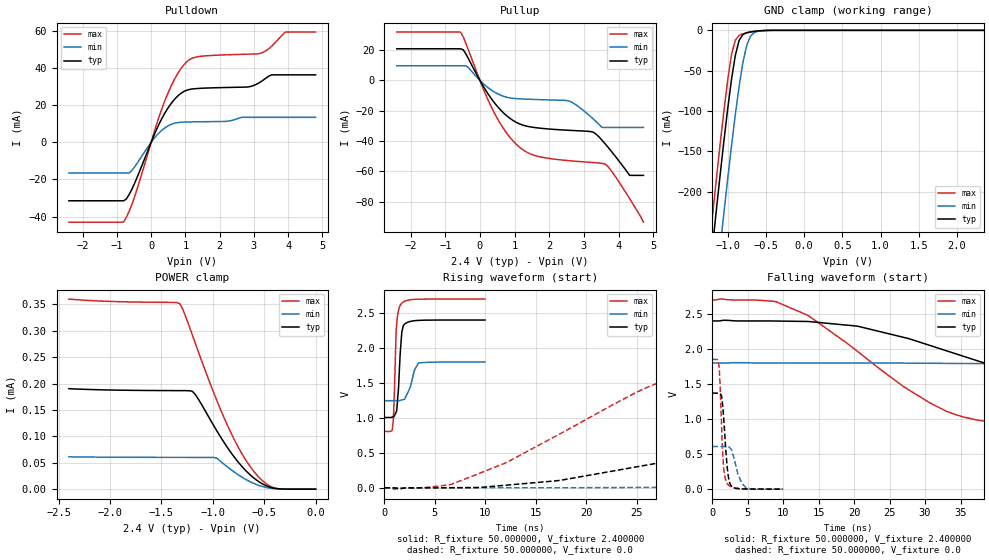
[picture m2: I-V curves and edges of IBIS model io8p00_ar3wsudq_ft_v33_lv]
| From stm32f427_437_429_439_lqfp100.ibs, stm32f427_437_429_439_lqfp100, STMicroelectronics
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|   Model io8p00_ar3wsudq_ft_v33_lv
[Model]  io8p00_ar3wsudq_ft_v33_lv
Model_type I/O
Polarity   Non-Inverting
Enable   Active-Low
Vinl =   0.720000V
Vinh =   1.680000V
Vmeas =  1.200000V
Cref =   50.000000pF
Rref =   100.000000M
Vref =   0.0V
C_comp   3.737300pF   3.690400pF   3.817400pF
[Temperature Range]   25.000000   0.125000k   -40.000000
[Pullup Reference]   2.400000V   1.800000V   2.700000V
[Pulldown Reference]   0.0V   0.0V   0.0V
[POWER Clamp Reference]   2.400000V   1.800000V   2.700000V
[GND Clamp Reference]   0.0V   0.0V   0.0V
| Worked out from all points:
|   slope of the pulldown table from 0 to 0.36 V, typ, clamps not added: 25 ohm
|   slope of the pullup table from 0 to 0.36 V, typ, clamps not added: 27.7 ohm
|   GND clamp passes 1 mA (typ) near -0.62 V on its own axis
|   rising waveform, R_fixture 50.000000, V_fixture 2.400000: 20-80 % time 349ps typ, 698ps min, 263ps max; typ from 1.01 V to 2.4 V
|   rising waveform, R_fixture 50.000000, V_fixture 0.0: 20-80 % time 30.9ns typ, 81.7ns min, 14.6ns max; typ from 0 V to 1.37 V
|   falling waveform, R_fixture 50.000000, V_fixture 2.400000: 20-80 % time 28.7ns typ, 81ns min, 15.9ns max; typ from 2.4 V to 1.01 V
|   falling waveform, R_fixture 50.000000, V_fixture 0.0: 20-80 % time 600ps typ, 1.08ns min, 461ps max; typ from 1.37 V to 0 V
[Pulldown]
|Voltage   I(typ)   I(min)   I(max)
-2.4V     -31.47mA   -16.45mA   -43.01mA
-800mV    -31.47mA   -16.45mA   -42.85mA
-480mV    -21.98mA   -13.17mA   -29.21mA
80mV      3.63mA     1.966mA    5.014mA
480mV     18.16mA    8.738mA    26.02mA
800mV     25.38mA    10.72mA    37.77mA
1.12V     28.53mA    11.02mA    44.6mA
2.8V      29.84mA    13.49mA    47.53mA
3.2V      32.65mA    13.49mA    48.04mA
3.52V     36.4mA     13.49mA    51.83mA
3.92V     36.4mA     13.49mA    59.44mA
4.8V      36.4mA     13.49mA    59.44mA
[Pullup]
|Voltage   I(typ)   I(min)   I(max)
-2.4V     20.89mA    9.661mA    31.89mA
-560mV    20.89mA    9.661mA    31.89mA
-400mV    17.28mA    9.661mA    24.06mA
320mV     -11.75mA   -6.207mA   -17.08mA
640mV     -20.52mA   -10.1mA    -30.35mA
960mV     -26.47mA   -11.82mA   -40.02mA
1.52V     -30.88mA   -12.51mA   -49.05mA
2.56V     -32.88mA   -13.52mA   -52.9mA
3.28V     -34.25mA   -25.62mA   -54.18mA
3.6V      -41.44mA   -30.99mA   -55.03mA
4.32V     -62.62mA   -30.99mA   -77.98mA
4.72V     -62.62mA   -30.99mA   -93.5mA
[GND_clamp]
|Voltage   I(typ)   I(min)   I(max)
-2.4V     -1.437A    -1.518A    -1.411A
-1.25V    -315.9mA   -407.2mA   -278.2mA
-1.2V     -270.1mA   -361.3mA   -232.1mA
-1.15V    -225mA     -316mA     -186.8mA
-1.1V     -180.9mA   -271.3mA   -142.7mA
-1.05V    -138.2mA   -227.5mA   -100.5mA
-950mV    -61.14mA   -143.6mA   -30.43mA
-900mV    -31.23mA   -104.7mA   -12.14mA
-850mV    -12.49mA   -69.4mA    -6.221mA
-750mV    -2.898mA   -18.35mA   -3.18mA
-600mV    -750.2uA   -1.218mA   -738.3uA
2.35V     0A         0A         0A
[POWER_clamp]
|Voltage   I(typ)   I(min)   I(max)
-2.4V     190.2uA    61.19uA    359.9uA
-1.32V    186.6uA    60.14uA    351.2uA
-1.29V    186.5uA    60.13uA    339.6uA
-1.2V     185.4uA    60.11uA    292.6uA
-1.17V    179.2uA    60.11uA    276.3uA
-960mV    110.2uA    58.62uA    167.5uA
-870mV    82.44uA    43.99uA    126.3uA
-750mV    50.58uA    26.92uA    78.64uA
-630mV    25.94uA    13.41uA    41.02uA
-510mV    9.22uA     4.527uA    14.97uA
-420mV    2.425uA    1.38uA     3.75uA
0V        0A         0A         0A
[Ramp]
| variable   typ   min   max
dV/dt_r  0.82266/30.92657n   0.36308/83.78730n   1.11084/14.58848n
dV/dt_f  0.83688/28.73017n   0.32688/81.44683n   1.13728/15.90715n
R_load = 50.000000
[Rising Waveform]
R_fixture= 50.000000
V_fixture= 2.400000
V_fixture_min= 1.800000
V_fixture_max= 2.700000
|time   V(typ)   V(min)   V(max)
0s        1.006V     1.247V     804.6mV
780.8ps   1.011V     1.247V     840.7mV
880.9ps   1.015V     1.247V     966.7mV
1.181ns   1.09V      1.247V     2.284V
1.381ns   1.4V       1.246V     2.53V
1.642ns   2.075V     1.253V     2.628V
1.722ns   2.226V     1.256V     2.64V
1.882ns   2.323V     1.262V     2.659V
3.383ns   2.395V     1.786V     2.699V
9.97ns    2.4V       1.8V       2.7V
[Rising Waveform]
R_fixture= 50.000000
V_fixture= 0.0
V_fixture_min= 0.0
V_fixture_max= 0.0
|time   V(typ)   V(min)   V(max)
0s        9.861nV    351.5nV    28.52nV
7.007ns   1.54mV     -65.12uV   70.14mV
12.01ns   36.61mV    -30.31uV   355mV
17.02ns   99.51mV    83.56uV    742.1mV
28.03ns   377mV      6.556mV    1.543V
39.04ns   686.7mV    29.19mV    1.767V
56.56ns   1.125V     88.61mV    1.83V
77.58ns   1.308V     182.7mV    1.85V
153.2ns   1.369V     510.1mV    1.852V
249.2ns   1.37V      609.1mV    1.852V
[Falling Waveform]
R_fixture= 50.000000
V_fixture= 2.400000
V_fixture_min= 1.800000
V_fixture_max= 2.700000
|time   V(typ)   V(min)   V(max)
0s        2.4V       1.8V       2.7V
9.009ns   2.399V     1.8V       2.673V
13.51ns   2.392V     1.8V       2.478V
20.52ns   2.324V     1.8V       1.962V
33.03ns   1.974V     1.794V     1.111V
43.54ns   1.63V      1.777V     913.4mV
58.06ns   1.27V      1.728V     852.7mV
82.58ns   1.087V     1.594V     820.6mV
156.2ns   1.012V     1.326V     804.6mV
249.2ns   1.006V     1.247V     804.6mV
[Falling Waveform]
R_fixture= 50.000000
V_fixture= 0.0
V_fixture_min= 0.0
V_fixture_max= 0.0
|time   V(typ)   V(min)   V(max)
0s        1.37V      609.1mV    1.852V
900.9ps   1.371V     609mV      1.797V
1.101ns   1.367V     608.9mV    1.451V
1.502ns   1.151V     608.6mV    432.4mV
1.702ns   858.8mV    608.7mV    214.5mV
2.062ns   351.7mV    608.5mV    87.34mV
2.683ns   44.82mV    566.8mV    32.76mV
3.584ns   8.565mV    225.2mV    11.26mV
4.785ns   2.572mV    15.07mV    3.432mV
9.97ns    9.861nV    351.5nV    28.52nV
